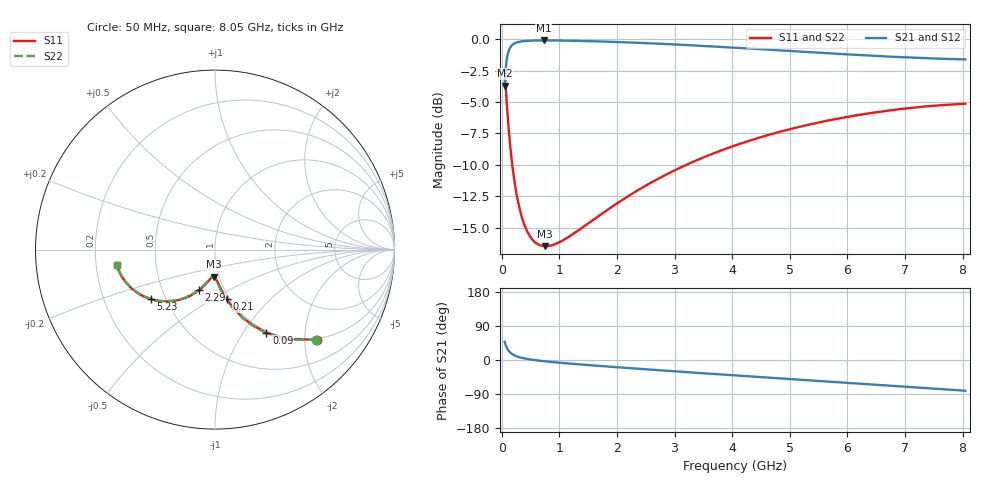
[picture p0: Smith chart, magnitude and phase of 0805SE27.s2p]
! AVX Thin Film Operation		Date: August 2001
! Description: Accu-P® Series, Thin Film, SMD, RF Capacitor
! Part Number: 08053J270FBT
! 50 MHz  -  8.05 GHz
! Serial Measurements
# mhz S db R 50
!	S11		S21		S12		S22
!	dB	Phase	dB	Phase	dB	Phase	dB	Phase
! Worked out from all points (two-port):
!   401 points, 50 MHz to 8.05 GHz, reference 50 ohm
!   highest |S21| = -0.10 dB at 730 MHz (marker M1); lowest = -3.7 dB at 50 MHz (marker M2)
!   |S21| within 3 dB of the highest: 58.39 MHz to end of sweep
!   lowest |S11| = -16.5 dB at 750 MHz (marker M3), VSWR 1.35, Z = 47.1 - j14.5 ohm
!   |S11| at or under -10 dB: 183.1 MHz to 3.207 GHz (3.024 GHz wide, 178 % of centre)
!   |S22| runs from -16.5 to -2.4 dB; largest |S21 - S12| = 0
!   S11 on the Smith chart (normalised r, x): 50 MHz: 0.97, -2.28; 90 MHz: 0.97, -1.28; 210 MHz: 0.97, -0.58; 2.29 GHz: 0.76, -0.37; 5.23 GHz: 0.42, -0.29; 8.05 GHz: 0.29, -0.07
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50  -2.42 -41.6  -3.69 48.4  -3.69 48.4  -2.42 -41.7
90  -5.28 -58.3  -1.53 31.6  -1.53 31.6  -5.28 -58.6
110  -6.53 -63.4  -1.09 26.4  -1.09 26.4  -6.53 -63.8
130  -7.64 -67.3  -0.82 22.4  -0.82 22.4  -7.64 -67.7
170  -9.49 -72.8  -0.52 16.9  -0.52 16.9  -9.49 -73.4
210  -10.96 -76.6  -0.37 13.1  -0.37 13.1  -10.96 -77.2
250  -12.13 -79.3  -0.28 10.3  -0.28 10.3  -12.13 -80.0
310  -13.48 -82.3  -0.20 7.2  -0.20 7.2  -13.48 -83.1
430  -15.18 -86.3  -0.14 3.1  -0.14 3.1  -15.18 -87.3
570  -16.13 -89.5  -0.11 -0.2  -0.11 -0.2  -16.13 -90.7
730  -16.47 -92.4  -0.10 -3.1  -0.10 -3.1  -16.47 -93.6
750  -16.48 -92.7  -0.10 -3.4  -0.10 -3.4  -16.48 -93.9
990  -16.18 -96.3  -0.11 -7.0  -0.11 -7.0  -16.18 -97.4
1390  -15.03 -101.4  -0.14 -12.1  -0.14 -12.1  -15.03 -102.5
2290  -12.23 -111.8  -0.27 -22.3  -0.27 -22.3  -12.23 -112.5
2730  -11.07 -116.5  -0.36 -27.0  -0.36 -27.0  -11.07 -117.2
3350  -9.71 -123.1  -0.50 -33.5  -0.50 -33.5  -9.71 -123.6
4050  -8.46 -130.3  -0.68 -40.7  -0.68 -40.7  -8.46 -130.7
5230  -6.91 -142.3  -1.00 -52.5  -1.00 -52.5  -6.91 -142.6
5390  -6.74 -143.9  -1.04 -54.1  -1.04 -54.1  -6.74 -144.2
6730  -5.67 -157.3  -1.39 -67.6  -1.39 -67.6  -5.67 -157.5
8050  -5.13 -170.9  -1.61 -81.1  -1.61 -81.1  -5.13 -171.0
